(* Logix 5000 AddOnInstructionDefinition export ACS_FAULTS_SAFETY_ACTIVE; software revision 20.01 *)

TYPE DriveFaults :
STRUCT
   Positive_Limit : BOOL;   // Positive Limit
   Negative_Limit : BOOL;   // Negative Limit
   E_Stop : BOOL;   // E Stop
   Position_Error : BOOL;   // Position Error
   Feedback_Error : BOOL;   // Feedback Error
   Over_Current : BOOL;   // Overcurrent
   Motor_Over_Temperature : BOOL;   // Motor Over Temperature
   Drive_Over_Temperature : BOOL;   // Drive Over Temperature
   Drive_Over_Voltage : BOOL;   // Drive Over Voltage
   Drive_Under_Voltage : BOOL;   // Drive Under Voltage
   Flash_Error : BOOL;   // Flash Error
   I2T_Limit : BOOL;   // I2T Limit Fault
   Short_Circuit : BOOL;   // Short Circuit Fault
   Watchdog_Reset : BOOL;   // Watchdog Reset
END_STRUCT
END_TYPE

ADD_ON_INSTRUCTION ACS_FAULTS_SAFETY_ACTIVE   (* revision 2.0, vendor Tolomatic, Inc *)
// True if ACS Drive contains any safety faults
VAR_IN_OUT
   DriveFaults : DINT; {required}   // ACS.I.FAULTS
END_VAR
VAR
   LocalFaults : DriveFaults; {access None}   // Local storage for faults
END_VAR

ROUTINE Logic   (* ladder *)
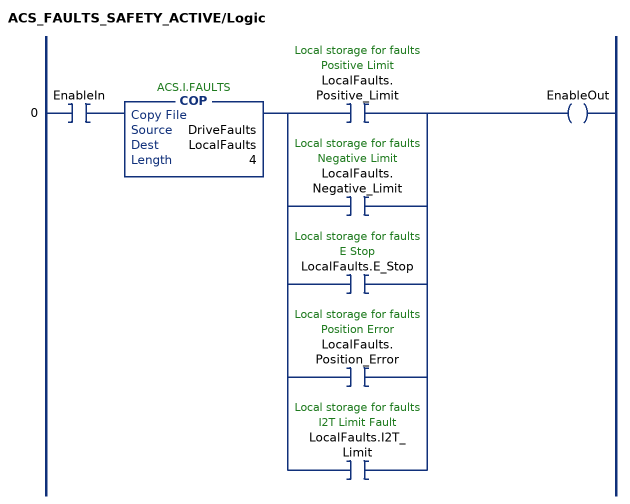
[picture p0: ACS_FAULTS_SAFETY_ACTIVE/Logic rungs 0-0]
   0: XIC(EnableIn)COP(DriveFaults,LocalFaults,4)[XIC(LocalFaults.Positive_Limit) ,XIC(LocalFaults.Negative_Limit) ,XIC(LocalFaults.E_Stop) ,XIC(LocalFaults.Position_Error) ,XIC(LocalFaults.I2T_Limit) ]OTE(EnableOut);
END_ROUTINE
END_ADD_ON_INSTRUCTION
